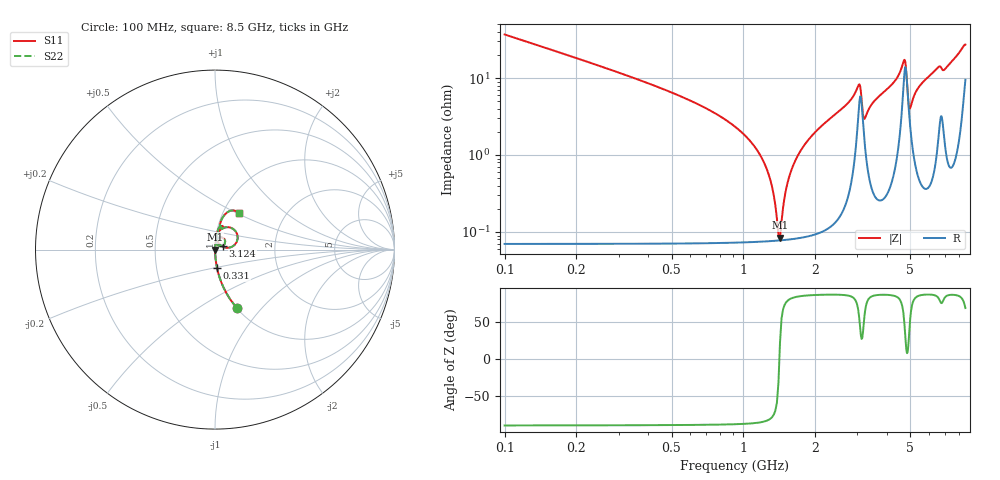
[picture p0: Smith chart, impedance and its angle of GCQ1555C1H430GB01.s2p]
!Murata Part Number: GCQ1555C1H430GB01
!These Parameters are Measured in Series Mode Connection
!Data Generated on Mar 13, 2026
!  o--ll--o
!Port1  Port2
!  o------o
!Operation Temp=25[degC], DC Bias Voltage=0[V]
!Freq. Start=100[MHz] Stop=9[GHz] 401[Steps]
# Hz S RI R 50
!Freq.(Hz) S11(Real) S11(Imag) S21(Real) S21(Imag) S12(Real) S12(Imag) S22(Real) S22(Imag)
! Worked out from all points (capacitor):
!   401 points, 100 MHz to 8.5 GHz, reference 50 ohm
!   read as one part in series: C = 43 pF near 142 MHz
!   lowest |Z| = 84.6 mohm at 1.423 GHz (marker M1)
!   series resonance near 1.414 GHz, so ESL is about 290 pH
!   S11 on the Smith chart (normalised r, x): 100 MHz: 1.00, -0.74; 331 MHz: 1.00, -0.21; 3.124 GHz: 1.09, +0.05; 8.5 GHz: 1.19, +0.51
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1e8  0.1199 -0.3239  0.8801 0.3239  0.8801 0.3239  0.1199 -0.3239
3.31e8  0.0118 -0.1045  0.9882 0.1045  0.9882 0.1045  0.0118 -0.1045
1.129e9  0.000889 -0.0121  0.9991 0.0121  0.9991 0.0121  0.000889 -0.0121
1.276e9  0.000789 -0.00552  0.9992 0.00552  0.9992 0.00552  0.000789 -0.00552
1.381e9  0.000773 -0.00128  0.9992 0.00128  0.9992 0.00128  0.000773 -0.00128
1.423e9  0.000777 0.000331  0.9992 -0.000331  0.9992 -0.000331  0.000777 0.000331
1.507e9  0.000803 0.00344  0.9992 -0.00344  0.9992 -0.00344  0.000803 0.00344
1.633e9  0.000877 0.00787  0.9991 -0.00787  0.9991 -0.00787  0.000877 0.00787
1.864e9  0.00112 0.0155  0.9989 -0.0155  0.9989 -0.0155  0.00112 0.0155
2.914e9  0.0118 0.0596  0.9882 -0.0596  0.9882 -0.0596  0.0118 0.0596
3.04e9  0.0419 0.0667  0.9581 -0.0667  0.9581 -0.0667  0.0419 0.0667
3.124e9  0.0455 0.0224  0.9545 -0.0224  0.9545 -0.0224  0.0455 0.0224
3.229e9  0.0134 0.0266  0.9866 -0.0266  0.9866 -0.0266  0.0134 0.0266
3.523e9  0.00547 0.0493  0.9945 -0.0493  0.9945 -0.0493  0.00547 0.0493
4.3e9  0.0144 0.089  0.9856 -0.089  0.9856 -0.089  0.0144 0.089
4.72e9  0.1143 0.1031  0.8857 -0.1031  0.8857 -0.1031  0.1143 0.1031
4.972e9  0.0272 0.0281  0.9728 -0.0281  0.9728 -0.0281  0.0272 0.0281
5.287e9  0.0109 0.0658  0.9891 -0.0658  0.9891 -0.0658  0.0109 0.0658
5.707e9  0.0119 0.0902  0.9881 -0.0902  0.9881 -0.0902  0.0119 0.0902
6.547e9  0.0337 0.1314  0.9663 -0.1314  0.9663 -0.1314  0.0337 0.1314
7.114e9  0.0275 0.1346  0.9725 -0.1346  0.9725 -0.1346  0.0275 0.1346
8.5e9  0.1335 0.2017  0.8665 -0.2017  0.8665 -0.2017  0.1335 0.2017
